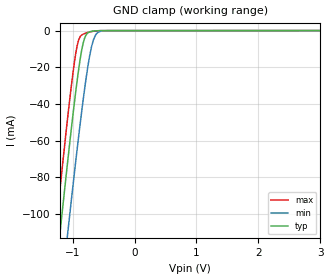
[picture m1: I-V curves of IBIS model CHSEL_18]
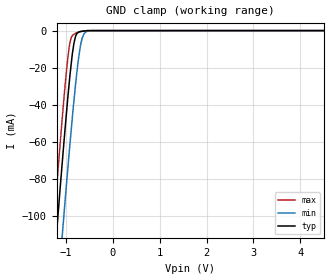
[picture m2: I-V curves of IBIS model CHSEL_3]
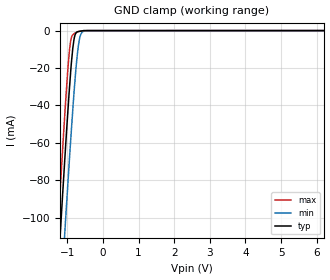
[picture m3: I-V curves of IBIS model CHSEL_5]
|Texas Instruments Incorporated
|12,10, 8 Bit 2 MSPS, Dual Channel, Unipolar Pseudo-differential
|   Ultra Low Power SAR Analog To Digital Converter
| Marketing part#   Digital Voltage Range   Package-type   #pins
|ADS7945SRTER   1.65 to 5.25V   QFN   16
|ADS7945SRTET   1.65 to 5.25V   QFN   16
|ADS7946SRTER   1.65 to 5.25V   QFN   16
|ADS7946SRTET   1.65 to 5.25V   QFN   16
|ADS7946SBRTER   1.65 to 5.25V   QFN   16
|ADS7946SBRTET   1.65 to 5.25V   QFN   16
|ADS7947SRTER   1.65 to 5.25V   QFN   16
|ADS7947SRTET   1.65 to 5.25V   QFN   16
|ADS7948SRTER   1.65 to 5.25V   QFN   16
|ADS7948SRTET   1.65 to 5.25V   QFN   16
|ADS7949SRTER   1.65 to 5.25V   QFN   16
|ADS7949SRTET   1.65 to 5.25V   QFN   16
[IBIS Ver]   4.0
[File name]   ads794x.ibs
[File Rev]   1.0
[Date]   05/19/2011
[Source]   Model genearted with SPECTRE and TISPICED
   Texas Instruments Incorporated.
   Analog-eLab, HPA
   12500 TI Blvd
   Dallas, TX -75243
   For Support e-mail: elab_ibis@list.ti.com
[Notes]   Revision History:
   1.0: 08/25/2010
   - Initial version of the model
   - Initial Model generated from simulations in TISPICED
   - Model not matched to measurements
   - Model names with a trailing
   _18 contains the model for 1.8V typ, 1.65V min,
   and 2V max operation.
   - Model names with a trailing
   _3 contains the model  for 3.3V typ, 3.0V min,
   and 3.6V max operation.
   - Model names with trailing
   _5 contains the model  for 5.0V typ, 4.75V min,
   and 5.25V maxoperation.
   - Ignore warnings related to typ, min and max values of ccomp,
   The device process of these products is CMOS. The ccomp
   values are based on PVT variations as seen in simulations
   2.0: 05/19/2011
   - Added ADS7945 and ADS7946 to this model.
[Disclaimer]
 This product is designed as an aid for customers of Texas Instruments.
 No warranties, either expressed or implied, with respect to this third
 party software (if any) or with respect to its fitness for any
 particular purpose is claimed by Texas Instruments or the author. The
 software (if any) is provided solely on an "as is" basis. The entire
 risk as to its quality and performance is with the customer
[Copyright] (C) Copyright 2010 Texas Instruments Incorporated.
   All rights reserved.
|   ADS7945, ADS7946
[Component]   ads7945_6
[Manufacturer] TI
[Package]   |WQFN - RTE package
| variable   typ   min   max
R_pkg  0.042266   0.000540  0.065360
L_pkg  0.707532nH 0.114770nH 1.090470nH
C_pkg  0.120390pF 0.069160pF 0.145430pF
[Pin] signal_name  model_name  R_pin  L_pin C_pin
1   GND   GND   0.06536  1.09047nH  0.13674pF
2   AVDD   POWER   0.05812  0.95811nH  0.14543pF
3   REF   TERM   0.05027  0.82268nH  0.13700pF
4   REFGND   GND   0.05682  0.94137nH  0.13137pF
5   AN0P   TERM   0.05741  0.94985nH  0.13267pF
6   AN0N   TERM   0.05199  0.84803nH  0.13715pF
7   AN1N   TERM   0.05496  0.90131nH  0.13980pF
8   AN1P   TERM   0.05236  0.85904nH  0.12385pF
9   NC   NC   0.00054  0.12002nH  0.06916pF
10  NC   NC   0.00054  0.11477nH  0.08199pF
11  CH_SEL   CHSEL   0.04738  0.76498nH  0.12888pF
12  PDEN   PDEN   0.04613  0.74897nH  0.11675pF
13  CS\   CS   0.04369  0.71116nH  0.11450pF
14  SCLK   SCLK   0.04355  0.70549nH  0.12599pF
15  SDO   SDO   0.04382  0.71024nH  0.12596pF
16  DVDD   POWER   0.04530  0.74105nH  0.11458pF
|   ADS7947, ADS7948, ADS7949
[Component]   ads7947_8_9
[Manufacturer] TI
[Package]   |WQFN - RTE package
| variable   typ   min   max
R_pkg  0.042266   0.000540  0.065360
L_pkg  0.707532nH 0.114770nH 1.090470nH
C_pkg  0.120390pF 0.069160pF 0.145430pF
[Pin] signal_name  model_name  R_pin  L_pin C_pin
1   VSS   POWER   0.06536  1.09047nH  0.13674pF
2   VDD   POWER   0.05812  0.95811nH  0.14543pF
3   REF+   TERM   0.05027  0.82268nH  0.13700pF
4   REF-   TERM   0.05682  0.94137nH  0.13137pF
5   Ch0+   TERM   0.05741  0.94985nH  0.13267pF
6   Ch0-   TERM   0.05199  0.84803nH  0.13715pF
7   Ch1-   TERM   0.05496  0.90131nH  0.13980pF
8   Ch1+   TERM   0.05236  0.85904nH  0.12385pF
9   NC   NC   0.00054  0.12002nH  0.06916pF
10  NC   NC   0.00054  0.11477nH  0.08199pF
11  CH_SEL   CHSEL   0.04738  0.76498nH  0.12888pF
12  PDEN   PDEN   0.04613  0.74897nH  0.11675pF
13  CS\   CS   0.04369  0.71116nH  0.11450pF
14  SCLK   SCLK   0.04355  0.70549nH  0.12599pF
15  SDO   SDO   0.04382  0.71024nH  0.12596pF
16  VBD   GND   0.04530  0.74105nH  0.11458pF
|   Model Selectors
|  Model names with a trailing
|   _18 contains the model for 1.8V typ, 1.65V min,
|   and 2V max operation.
|  Model names with a trailing
|   _3 contains the model  for 3.3V typ, 3.0V min,
|   and 3.6V max operation..
|  Model names with trailing
|   _5 contains the model  for 5.0V typ, 4.75V min,
|   and 5.25V maxoperation.
[Model Selector]  CHSEL
CHSEL_18  1.8V digital input
CHSEL_3   3.3V digital input
CHSEL_5   5V   digital input
[Model Selector]  PDEN
PDEN_18  1.8V digital input
PDEN_3   3.3V digital input
PDEN_5   5V   digital input
[Model Selector]  CS
CS_18  1.8V digital input
CS_3   3.3V digital input
CS_5   5V   digital input
[Model Selector]  SCLK
SCLK_18  1.8V digital input
SCLK_3   3.3V digital input
SCLK_5   5V   digital input
[Model Selector]  SDO
SDO_18 1.8V digital output
SDO_3  3.3V digital output
SDO_5  5V digital output
|   TERM Model
[Model] TERM
Model_type Terminator
C_comp   1e-20   1e-20   1e-20
| variable   typ   min   max
[Voltage Range]   2.7V   2.0V   5.25V
[POWER Clamp Reference]  2.7V   2.0V   5.25V
[GND Clamp Reference]   0.0V   0.0V   0.0V
|Operating Temperature
[Temperature Range]   27   125   -40
| Models and submodels in the file (16): TERM (Terminator), CHSEL_18 (Input), CHSEL_3 (Input), CHSEL_5 (Input), PDEN_18 (Input), PDEN_3 (Input), PDEN_5 (Input), CS_18 (Input), CS_3 (Input), CS_5 (Input), SCLK_18 (Input), SCLK_3 (Input), SCLK_5 (Input), SDO_18 (3-state), SDO_3 (3-state), SDO_5 (3-state)
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|   CHSEL 1.8V Model
[Model] CHSEL_18
Model_type   Input
Vinl = 0.54
Vinh = 1.26
|   typ   min   max
|   (Nom PVT)   (Fast PVT)  (Slow PVT)
C_comp   9.3674890e-13  7.6575000e-13   1.1129200e-12
| POWER = 1.8V
[Model Spec]
Vinl   0.54   0.495   0.6
Vinh   1.26   1.155   1.4
|Vinl = 0.3 X DVDD
|Vinh = 0.7 X DVDD
[Voltage Range]   1.8   1.65   2
[Temperature Range]   27   125   -40
[Power Clamp Reference]   1.8   1.65   2
[GND Clamp Reference]   0   0   0
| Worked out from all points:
|   GND clamp passes 1 mA (typ) near -0.74 V on its own axis
[GND Clamp]
|   Voltage   I(typ)   I(min)   I(max)
-1.8V     -308.6mA   -345.1mA   -287mA
-1.276V   -134.2mA   -173.1mA   -110.5mA
-1.208V   -112.2mA   -151.4mA   -88.18mA
-1.088V   -74.28mA   -113.5mA   -50.27mA
-1.055V   -64.08mA   -103.3mA   -40.24mA
-939.6mV  -30.91mA   -68.63mA   -10.72mA
-901.1mV  -21.17mA   -57.6mA    -5.101mA
-834.8mV  -7.837mA   -39.33mA   -2.022mA
-779.5mV  -2.233mA   -25.65mA   -1.343mA
-691.1mV  -411.9uA   -8.484mA   -566.8uA
-562.9mV  -38.2uA    -510.7uA   -72.75uA
3.595V    0A         0A         0A
[POWER Clamp]
|   SCR cell for ESD function. Effects occurr above VDD x 2
|   Voltage   I(typ)   I(min)   I(max)
-1.8V     0A         0A         0A
0V        0A         0A         0A
3.6V      0A         0A         0A
|   CHSEL 3.3V Model
[Model] CHSEL_3
Model_type   Input
Vinl = 0.99
Vinh = 2.31
|   typ   min   max
|   (Nom PVT)   (Fast PVT)  (Slow PVT)
C_comp   8.5690020e-13   7.0889300e-13   1.0102340e-12
|POWER = 3.3v
[Model Spec]
Vinl   0.99   0.9   1.08
Vinh   2.31   2.1   2.52
|Vinl = 0.3 X DVDD
|Vinh = 0.7 X DVDD
[Voltage Range]   3.3   3   3.6
[Temperature Range]   27   125   -40
[Power Clamp Reference]   3.3   3   3.6
[GND Clamp Reference]   0   0   0
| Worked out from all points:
|   GND clamp passes 1 mA (typ) near -0.74 V on its own axis
[GND Clamp]
|   Voltage   I(typ)   I(min)   I(max)
-3.3V     -821.8mA   -851.7mA   -804.8mA
-1.274V   -133.6mA   -172.6mA   -109.8mA
-1.191V   -106.6mA   -145.9mA   -82.69mA
-1.091V   -75.13mA   -114.5mA   -51.13mA
-1.035V   -58.06mA   -97.15mA   -34.43mA
-925mV    -27.16mA   -64.45mA   -8.184mA
-829.4mV  -6.955mA   -38.07mA   -2.026mA
-723.5mV  -668.5uA   -13.78mA   -835.8uA
-677.9mV  -498.6uA   -6.75mA    -472.6uA
-614.2mV  -260.7uA   -1.748mA   -217uA
-440.3mV  -20.36uA   -24.09uA   -20.25uA
6.59V     0A         0A         0A
[POWER Clamp]
|   SCR cell for ESD function. Effects occurr above VDD x 2
|   Voltage   I(typ)   I(min)   I(max)
-3.3V     0A         0A         0A
0V        0A         0A         0A
6.6V      0A         0A         0A
|   CHSEL 5V Model
[Model] CHSEL_5
Model_type   Input
Vinl = 1.5
Vinh = 3.5
|   typ   min   max
C_comp   7.9739720e-13   6.6899650e-13   9.2619770e-13
|   (Nom PVT)   (Fast PVT)  (Slow PVT)
|POWER = 5V
[Model Spec]
Vinl   1.5   1.35   1.65
Vinh   3.5   3.15   3.85
|Vinl = 0.3 X DVDD
|Vinh = 0.7 X DVDD
[Voltage Range]   5   4.75   5.25
[Temperature Range]   27   125   -40
[Power Clamp Reference]   5   4.75   5.25
[GND Clamp Reference]   0   0   0
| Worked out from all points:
|   GND clamp passes 1 mA (typ) near -0.74 V on its own axis
[GND Clamp]
|   Voltage   I(typ)   I(min)   I(max)
-5V       -1.409A    -1.433A    -1.396A
-1.296V   -140.7mA   -179.6mA   -116.9mA
-1.257V   -128.1mA   -167.2mA   -104.3mA
-1.194V   -107.9mA   -147mA     -83.76mA
-1.085V   -73.59mA   -112.8mA   -49.43mA
-1.047V   -61.81mA   -100.9mA   -38.07mA
-935.3mV  -29.91mA   -67.37mA   -9.922mA
-810.2mV  -4.597mA   -33.02mA   -1.71mA
-721.3mV  -642uA     -13.4mA    -812.8uA
-610.8mV  -260.5uA   -1.615mA   -227.9uA
-431.8mV  -16.09uA   -19.14uA   -15.55uA
9.985V    0A         0A         0A
[POWER Clamp]
|   SCR cell for ESD function. Effects occurr above VDD x 2
|   Voltage   I(typ)   I(min)   I(max)
-5V       0A         0A         0A
0V        0A         0A         0A
10V       0A         0A         0A
